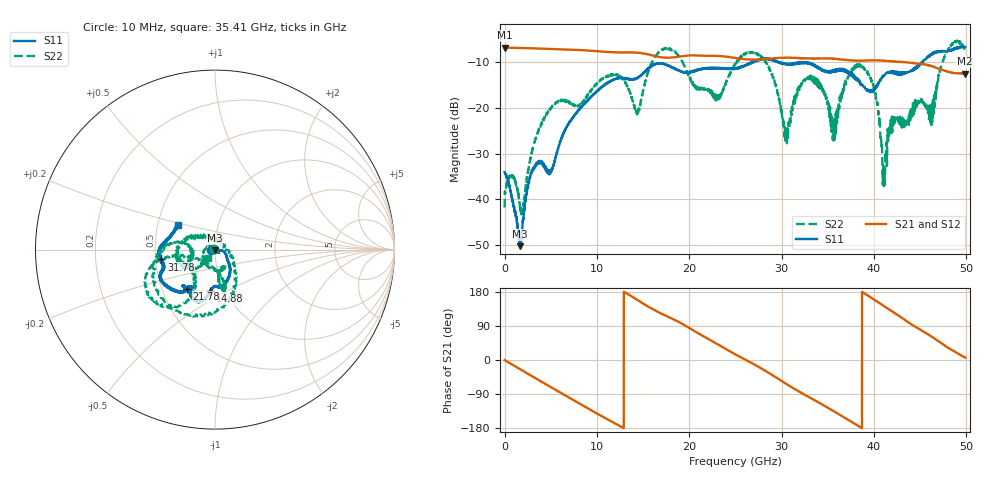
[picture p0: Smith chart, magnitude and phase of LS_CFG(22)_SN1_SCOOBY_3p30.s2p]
!Keysight Technologies,N5245B,MY58422026,A.13.80.08
!Date: Thursday, March 19, 2020 23:33:37
!Correction: S11(Full 2 Port(1,2))
!S21(Full 2 Port(1,2))
!S12(Full 2 Port(1,2))
!S22(Full 2 Port(1,2))
!S2P File: Measurements: S11, S21, S12, S22:
# Hz S DB R 50.0
!freq dBS11 angS11 dBS21 angS21 dBS12 angS12 dBS22 angS22
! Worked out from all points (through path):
!   4991 points, 10 MHz to 49.91 GHz, reference 50 ohm
!   highest |S21| = -6.79 dB at 10 MHz (marker M1); lowest = -12.5 dB at 49.83 GHz (marker M2)
!   group delay of S21, straight-line fit = 39.3 ps
!   lowest |S11| = -50.3 dB at 1.68 GHz (marker M3), VSWR 1.01, Z = 49.9 - j0.297 ohm
!   |S11| at or under -10 dB: start of sweep to 26.79 GHz; 29.82 GHz to 31.96 GHz (2.143 GHz wide, 6.94 % of centre); 32.7 GHz to 45.16 GHz (12.45 GHz wide, 32 % of centre)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
!   |S22| runs from -43.8 to -5.3 dB; largest |S21 - S12| = 0.0044
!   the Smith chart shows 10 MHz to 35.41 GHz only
!   S11 on the Smith chart (normalised r, x): 10 MHz: 0.96, -0.01; 14.88 GHz: 0.85, -0.42; 21.78 GHz: 0.67, -0.32; 31.78 GHz: 0.54, -0.06; 35.41 GHz: 0.64, +0.19
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1e7  -34.06 -170.8  -6.79 -0.3  -6.78 -0.3  -41.82 170.0
1.68e9  -50.28 -103.6  -6.88 -24.2  -6.88 -24.2  -41.90 -31.0
2.91e9  -34.23 -28.7  -6.97 -41.7  -6.97 -41.7  -30.06 136.1
4.42e9  -32.74 -37.7  -7.07 -63.1  -7.07 -63.1  -21.66 -145.0
8.33e9  -19.91 -43.0  -7.37 -118.1  -7.37 -118.0  -19.06 -72.4
1.488e10  -12.63 -96.5  -8.04 150.9  -8.04 151.0  -17.33 -161.1
1.665e10  -10.31 -108.5  -8.81 126.4  -8.80 126.4  -7.94 -160.4
2.178e10  -11.38 -125.6  -8.60 59.5  -8.60 59.6  -15.83 -154.5
2.496e10  -11.44 -129.6  -9.05 15.4  -9.04 15.5  -10.60 -177.9
2.819e10  -9.33 -149.6  -9.32 -27.7  -9.32 -27.7  -9.83 -84.6
3.05e10  -10.42 -161.9  -9.03 -62.9  -9.03 -62.7  -25.54 48.9
3.178e10  -10.37 -169.6  -9.12 -81.9  -9.12 -81.6  -16.30 156.4
3.328e10  -10.36 175.8  -9.19 -102.3  -9.19 -102.0  -13.27 -161.8
3.541e10  -12.20 146.4  -9.19 -131.8  -9.15 -131.4  -24.29 -130.5
3.85e10  -14.72 112.6  -9.68 -176.7  -9.64 -176.9  -10.83 -152.0
4.018e10  -15.77 70.8  -9.60 156.7  -9.58 156.5  -16.88 -92.3
4.106e10  -12.85 51.5  -9.67 142.5  -9.69 142.4  -35.95 62.4
4.16e10  -12.13 46.4  -9.77 134.0  -9.79 133.8  -24.46 131.9
4.675e10  -7.64 -19.2  -11.23 53.5  -11.25 53.6  -15.45 -137.6
4.841e10  -7.27 -37.6  -12.31 27.2  -12.34 27.2  -6.09 -62.8
4.983e10  -6.64 -43.5  -12.50 6.9  -12.51 7.0  -7.09 -13.3
4.991e10  -6.72 -43.1  -12.45 6.0  -12.47 5.9  -7.57 -14.1
